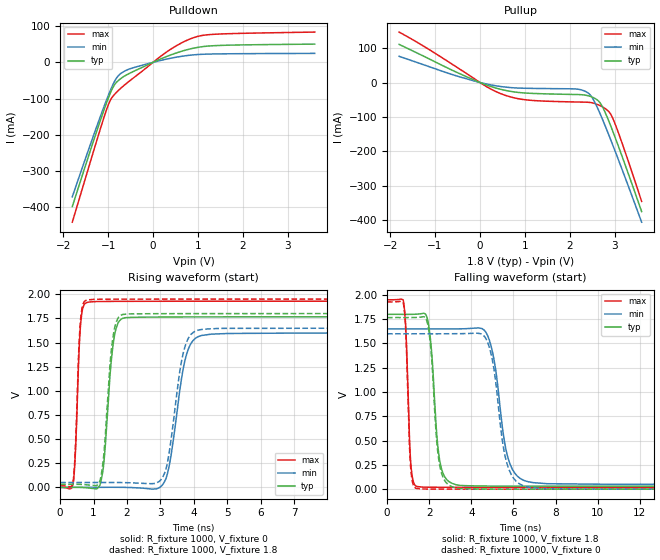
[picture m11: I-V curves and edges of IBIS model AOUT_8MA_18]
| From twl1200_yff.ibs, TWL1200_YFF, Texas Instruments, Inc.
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[Model]   AOUT_8MA_18
Model_type  Output
Vref =   1.8
Rref =   1M
Cref =   15p
Vmeas =   0.9
| variable   typ   min   max
C_comp   4.37pF   2.85pF   5.56pF
| C_pullup   4.60pF   2.85pF   5.56pF
| C_pulldown   4.13pF   3.05pF   5.23pF
[Temperature Range]   40   100   -40
| Ambient temperature   25   85   -40
[Voltage range]   1.8   1.65   1.95
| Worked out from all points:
|   slope of the pulldown table from 0 to 0.27 V, typ, clamps not added: 18.6 ohm
|   slope of the pullup table from 0 to 0.27 V, typ, clamps not added: 21.1 ohm
|   rising waveform, R_fixture 1000, V_fixture 0: 20-80 % time 229ps typ, 400ps min, 125ps max; typ from 0 V to 1.77 V
|   falling waveform, R_fixture 1000, V_fixture 1.8: 20-80 % time 340ps typ, 604ps min, 180ps max; typ from 1.8 V to 0.031 V
|   rising waveform, R_fixture 1000, V_fixture 1.8: 20-80 % time 223ps typ, 381ps min, 122ps max; typ from 0.031 V to 1.8 V
|   falling waveform, R_fixture 1000, V_fixture 0: 20-80 % time 333ps typ, 584ps min, 173ps max; typ from 1.77 V to 0 V
[Pulldown]
| AOUT_8MA_18
|   Voltage   I(typ)   I(min)   I(max)
-1.8V     -398.9mA   -371.9mA   -441.9mA
-1.365V   -231.8mA   -215.8mA   -261.5mA
-1.09V    -130.5mA   -121.4mA   -150.7mA
-975mV    -91.89mA   -84.7mA    -111mA
-880mV    -66.2mA    -57.88mA   -91.81mA
-770mV    -50mA      -36.46mA   -77.27mA
-605mV    -35.67mA   -22.46mA   -59.46mA
110mV     6.157mA    3.454mA    11.02mA
630mV     30.38mA    16.52mA    53.46mA
1.09V     43.16mA    22.18mA    74.23mA
1.695V    47.46mA    23.65mA    79.22mA
3.6V      50.33mA    24.73mA    83.6mA
[Pullup]
| AOUT_8MA_18
|   Voltage   I(typ)   I(min)   I(max)
-1.8V     110.8mA    76.17mA    146.6mA
-310mV    17.42mA    11.3mA     27.04mA
160mV     -7.986mA   -4.814mA   -13.09mA
510mV     -21.33mA   -12.47mA   -34.73mA
1.095V    -31.23mA   -16.97mA   -51.35mA
2.135V    -34.9mA    -18.85mA   -56.64mA
2.4V      -38.24mA   -29.69mA   -57.46mA
2.515V    -43.37mA   -47.5mA    -59.6mA
2.675V    -59.17mA   -90.8mA    -67.32mA
2.92V     -129.1mA   -169.5mA   -94.21mA
3.135V    -204.1mA   -242.6mA   -165.3mA
3.6V      -375.3mA   -406.2mA   -345.8mA
[Ramp]
| AOUT_8MA_18
| variable   typ   min   max
dV/dt_r   1.07/2.43E-10   0.97/4.13E-10   1.17/1.26E-10
dV/dt_f   1.07/3.47E-10   0.97/6.11E-10   1.16/1.98E-10
R_load = 1000
[Rising Waveform]
| AOUT_8MA_18
R_fixture =   1000
C_fixture =   0
L_fixture =   0
V_fixture =   0
V_fixture_min = 0
V_fixture_max = 0
|   Time   V(typ)   V(min)   V(max)
0s        7.131nV    37.03nV    538.1pV
400ps     880.7uV    -1.377uV   64.37mV
660ps     -241.3uV   -22.48uV   1.83V
1.095ns   -15.89mV   28.06uV    1.924V
1.64ns    1.599V     1.017mV    1.926V
2.15ns    1.761V     -1.95mV    1.927V
3.165ns   1.764V     89.94mV    1.927V
3.925ns   1.765V     1.497V     1.927V
5.03ns    1.766V     1.594V     1.928V
238ns     1.766V     1.6V       1.928V
[Falling Waveform]
| AOUT_8MA_18
R_fixture =   1000
C_fixture =   0
L_fixture =   0
V_fixture =   1.8
V_fixture_min = 1.65
V_fixture_max = 1.95
|   Time   V(typ)   V(min)   V(max)
0s        1.8V       1.65V      1.95V
780ps     1.799V     1.65V      1.934V
1.145ns   1.8V       1.65V      221.1mV
1.655ns   1.807V     1.65V      21.61mV
2.575ns   218.3mV    1.65V      19.46mV
3.68ns    36.34mV    1.651V     19.06mV
4.85ns    31.94mV    1.538V     18.92mV
5.945ns   31.4mV     206.1mV    18.86mV
7.6ns     31.15mV    56.19mV    18.83mV
238ns     31.03mV    50.12mV    18.81mV
[Rising Waveform]
| AOUT_8MA_18
R_fixture =   1000
C_fixture =   0
L_fixture =   0
V_fixture =   1.8
V_fixture_min = 1.65
V_fixture_max = 1.95
|   Time   V(typ)   V(min)   V(max)
0s        31.03mV    50.12mV    18.81mV
390ps     31.76mV    50.12mV    71.63mV
625ps     31mV       50.11mV    1.784V
1.045ns   18.38mV    50.13mV    1.947V
1.62ns    1.636V     50.67mV    1.949V
2.055ns   1.797V     48.38mV    1.949V
3.065ns   1.799V     102.8mV    1.95V
3.785ns   1.799V     1.507V     1.95V
4.785ns   1.8V       1.646V     1.95V
238ns     1.8V       1.65V      1.95V
[Falling Waveform]
| AOUT_8MA_18
R_fixture =   1000
C_fixture =   0
L_fixture =   0
V_fixture =   0
V_fixture_min = 0
V_fixture_max = 0
|   Time   V(typ)   V(min)   V(max)
0s        1.766V     1.6V       1.928V
775ps     1.766V     1.6V       1.917V
1.135ns   1.767V     1.6V       186.8mV
1.61ns    1.771V     1.6V       2.57mV
2.56ns    185.7mV    1.6V       579.4uV
3.605ns   5.143mV    1.601V     240.6uV
4.815ns   818.9uV    1.489V     98.68uV
5.895ns   349.4uV    151.2mV    47uV
7.455ns   121.6uV    5.685mV    16.66uV
238ns     14.33nV    40.6nV     6.149nV
